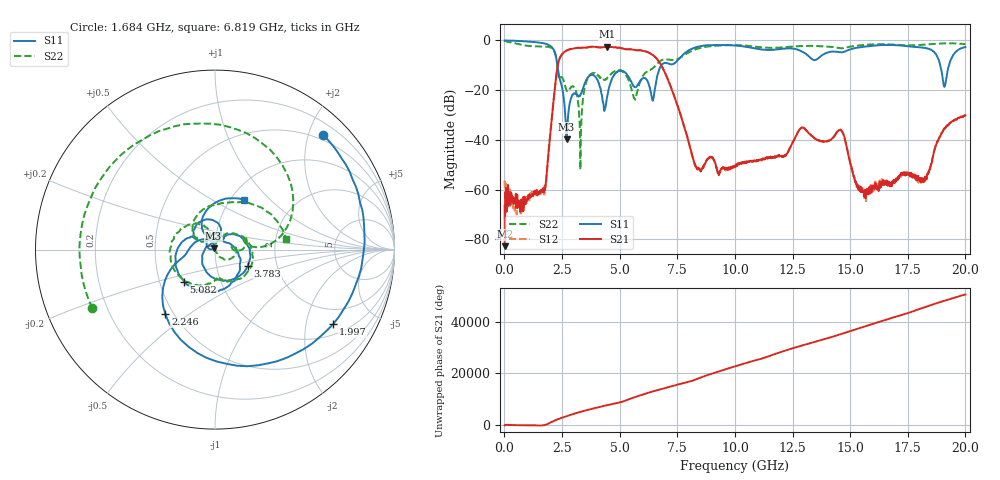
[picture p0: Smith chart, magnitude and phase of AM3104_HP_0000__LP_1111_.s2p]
!Created with skrf (http://scikit-rf.org).
# Hz S RI R 50.0
!freq ReS11 ImS11 ReS21 ImS21 ReS12 ImS12 ReS22 ImS22
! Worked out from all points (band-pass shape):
!   1601 points, 10 MHz to 20 GHz, reference 50 ohm
!   highest |S21| = -2.43 dB at 4.458 GHz (marker M1); lowest = -82.7 dB at 22.49 MHz (marker M2)
!   |S21| within 3 dB of the highest: 2.511 GHz to 6.36 GHz (3.849 GHz wide, 86.8 % of centre)
!   lowest |S11| = -39.8 dB at 2.696 GHz (marker M3), VSWR 1.02, Z = 49.2 + j0.635 ohm
!   |S11| at or under -10 dB: 2.302 GHz to 6.808 GHz (4.507 GHz wide, 98.9 % of centre); 18.91 GHz to 19.29 GHz (378.4 MHz wide, 1.98 % of centre)
!   |S22| runs from -51.9 to -0.1 dB; largest |S21 - S12| = 0.0087
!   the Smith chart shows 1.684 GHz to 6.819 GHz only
!   S11 on the Smith chart (normalised r, x): 1.684 GHz: 0.40, +2.25; 1.997 GHz: 1.36, -2.87; 2.246 GHz: 0.45, -0.41; 3.783 GHz: 1.42, -0.26; 5.082 GHz: 0.67, -0.25; 6.819 GHz: 1.14, +0.71
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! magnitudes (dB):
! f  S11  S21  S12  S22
! 10 MHz  0.0  -66.5  -56.4  -0.1
! 22.49 MHz  0.0  -82.7  -59.5  -0.1
! 1.684 GHz  -1.1  -59.3  -60.0  -2.4
! 1.997 GHz  -2.2  -37.0  -37.0  -2.8
! 2.246 GHz  -6.9  -14.4  -14.4  -6.9
! 2.696 GHz  -39.8  -4.0  -4.0  -20.0
! 3.346 GHz  -21.0  -2.9  -2.9  -31.1
! 3.783 GHz  -13.8  -2.5  -2.5  -13.3
! 4.458 GHz  -22.7  -2.4  -2.4  -15.1
! 5.082 GHz  -12.1  -3.1  -3.1  -12.2
! 5.657 GHz  -18.8  -3.8  -3.8  -23.7
! 6.682 GHz  -12.6  -8.2  -8.2  -8.9
! 6.819 GHz  -9.9  -10.2  -10.2  -7.9
! 8.331 GHz  -2.7  -51.2  -51.1  -3.4
! 10.01 GHz  -2.0  -50.6  -50.5  -1.8
! 13.34 GHz  -7.4  -38.5  -38.4  -2.2
! 14.63 GHz  -4.7  -36.3  -36.3  -3.1
! 15.63 GHz  -2.5  -62.0  -62.0  -1.8
! 16.68 GHz  -1.8  -56.7  -58.0  -1.5
! 18.24 GHz  -3.0  -56.0  -55.9  -1.6
! 19.1 GHz  -18.5  -35.4  -35.3  -1.2
! 20 GHz  -2.6  -30.1  -30.2  -1.5
